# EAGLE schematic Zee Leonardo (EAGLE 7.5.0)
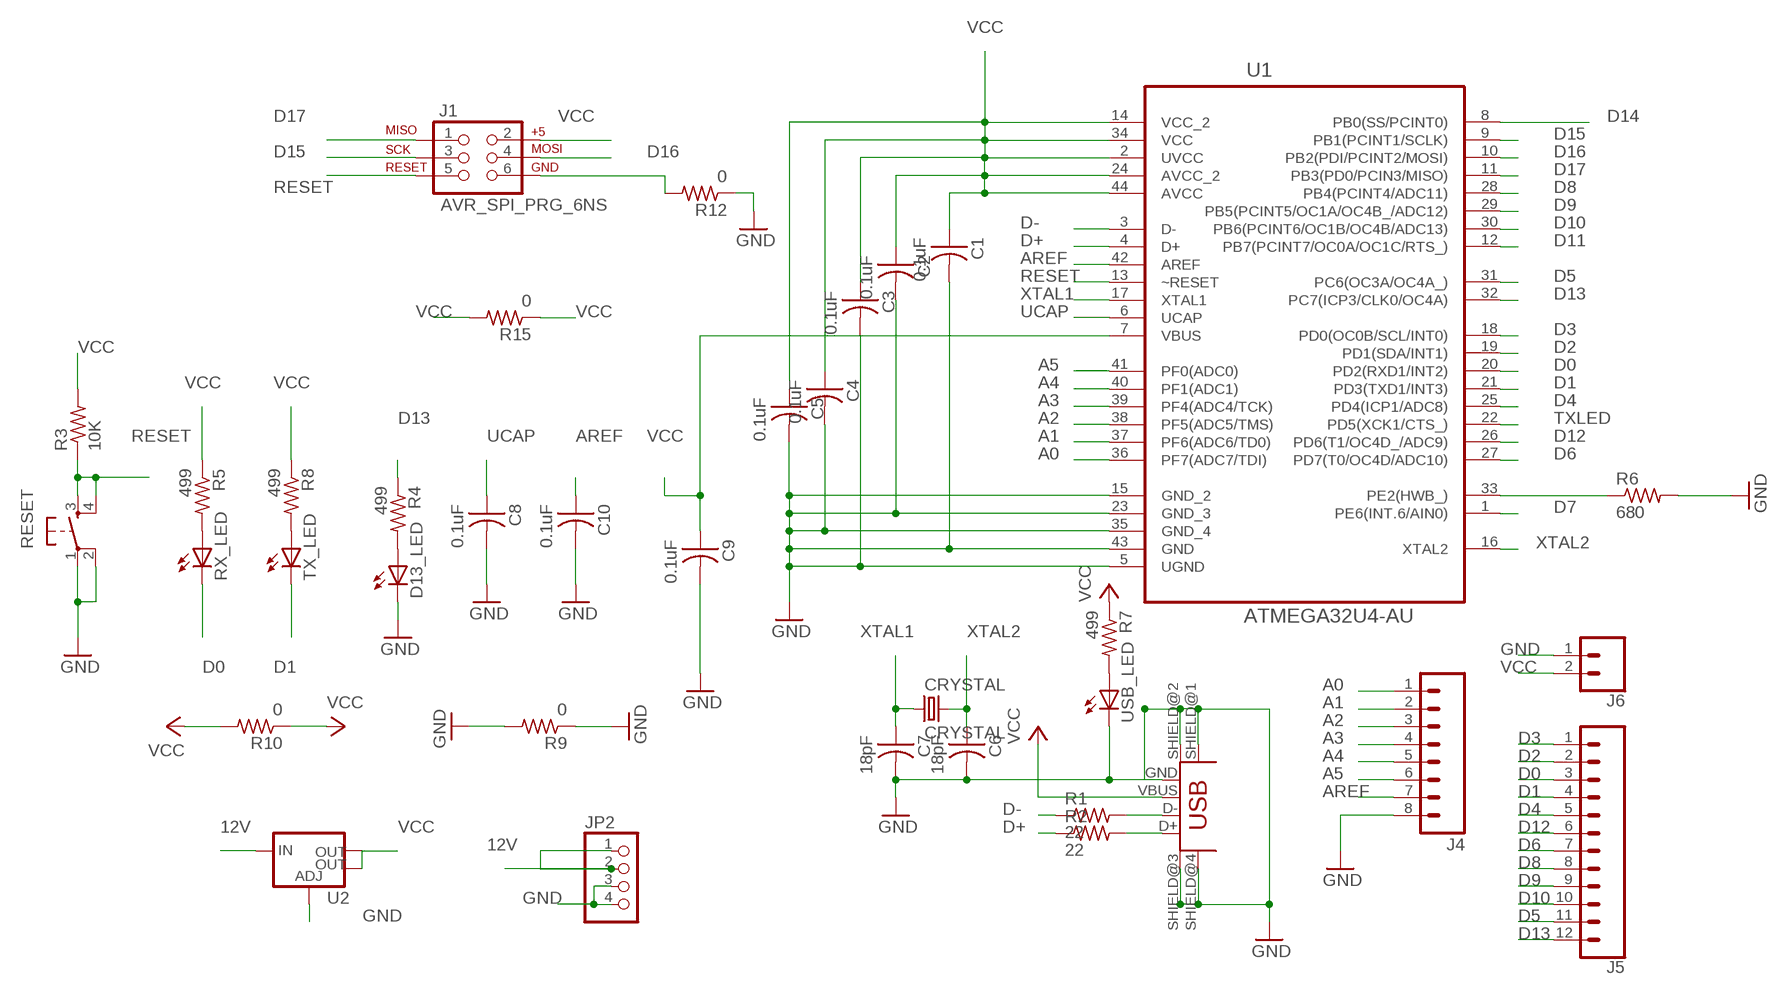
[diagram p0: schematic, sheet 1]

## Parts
C1  0.1uF  CAP-US1206FAB  [C1206FAB]
C2  0.1uF  CAP-US1206FAB  [C1206FAB]
C3  0.1uF  CAP-US1206FAB  [C1206FAB]
C4  0.1uF  CAP-US1206FAB  [C1206FAB]
C5  0.1uF  CAP-US1206FAB  [C1206FAB]
C6  18pF  CAP-US1206FAB  [C1206FAB]
C7  18pF  CAP-US1206FAB  [C1206FAB]
C8  0.1uF  CAP-US1206FAB  [C1206FAB]
C9  0.1uF  CAP-US1206FAB  [C1206FAB]
C10  0.1uF  CAP-US1206FAB  [C1206FAB]
CRYSTAL  CRYSTAL  [2-SMD-5X3MM]
D13_LED  LED1206  [1206]
J1  AVR_SPI_PRG_6NS  [2X3-NS]
J4  M08NO_SILK  [1X08_PIN1_NO_SILK]
J5  CONN_12NO_SILK  [1X12_NO_SILK]
J6  CONN_021X02_NO_SILK  [1X02_NO_SILK]
JP2  PINHD-1X4  [1X04]
R1  22  RES-US1206FAB  [R1206FAB]
R2  22  RES-US1206FAB  [R1206FAB]
R3  10K  RES-US1206FAB  [R1206FAB]
R4  499  RESISTOR1206  [1206]
R5  499  RESISTOR1206  [1206]
R6  680  RES-US1206FAB  [R1206FAB]
R7  499  RESISTOR1206  [1206]
R8  499  RESISTOR1206  [1206]
R9  0  RES-US1206FAB  [R1206FAB]
R10  0  RES-US1206FAB  [R1206FAB]
R12  0  RES-US1206FAB  [R1206FAB]
R15  0  RES-US1206FAB  [R1206FAB]
RESET  6MM_SWITCH6MM_SWITCH  [6MM_SWITCH]
RX_LED  LED1206  [1206]
TX_LED  LED1206  [1206]
U1  ATMEGA32U4-AU  [QFP80P1200X1200X120-44N]
U2  V_REG_LM1117SOT223  [SOT223]
USB_LED  LED1206  [1206]
USB_UPLOAD  USB_MINIB  [USB_MINIB]

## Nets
12V: JP2.1 JP2.2 U2.3(IN)
A0: J4.1 U1.36(PF7(ADC7/TDI))
A1: J4.2 U1.37(PF6(ADC6/TD0))
A2: J4.3 U1.38(PF5(ADC5/TMS))
A3: J4.4 U1.39(PF4(ADC4/TCK))
A4: J4.5 U1.40(PF1(ADC1))
A5: J4.6 U1.41(PF0(ADC0))
AREF: C10.1 J4.7 U1.42(AREF)
D0: J5.3 RX_LED.2(C) U1.20(PD2(RXD1/INT2))
D1: J5.4 TX_LED.2(C) U1.21(PD3(TXD1/INT3))
D2: J5.2 U1.19(PD1(SDA/INT1))
D3: J5.1 U1.18(PD0(OC0B/SCL/INT0))
D4: J5.5 U1.25(PD4(ICP1/ADC8))
D5: J5.11 U1.31(PC6(OC3A/OC4A_))
D6: J5.7 U1.27(PD7(T0/OC4D/ADC10))
D7: U1.1(PE6(INT.6/AIN0))
D8: J5.8 U1.28(PB4(PCINT4/ADC11))
D9: J5.9 U1.29(PB5(PCINT5/OC1A/OC4B_/ADC12))
D10: J5.10 U1.30(PB6(PCINT6/OC1B/OC4B/ADC13))
D11: U1.12(PB7(PCINT7/OC0A/OC1C/RTS_))
D12: J5.6 U1.26(PD6(T1/OC4D_/ADC9))
D13: J5.12 R4.1 U1.32(PC7(ICP3/CLK0/OC4A))
D14: U1.8(PB0(SS/PCINT0))
D15: J1.3 U1.9(PB1(PCINT1/SCLK))
D16: J1.4 U1.10(PB2(PDI/PCINT2/MOSI))
D17: J1.1 U1.11(PB3(PD0/PCIN3/MISO))
D+: R2.1 U1.4(D+)
D-: R1.1 U1.3(D-)
GND: C1.2 C2.2 C3.2 C4.2 C5.2 C6.2 C7.2 C8.2 C9.2 C10.2 D13_LED.2(C) J4.8 J6.1 JP2.3 JP2.4 R6.2 R9.1 R9.2 R12.1 RESET.1(P) RESET.2(P1) U1.5(UGND) U1.15(GND_2) U1.23(GND_3) U1.35(GND_4) U1.43(GND) U2.1(ADJ) USB_LED.2(C) USB_UPLOAD.GND USB_UPLOAD.SHIELD@1(SHIELD) USB_UPLOAD.SHIELD@2(SHIELD1) USB_UPLOAD.SHIELD@3(SHIELD2) USB_UPLOAD.SHIELD@4(SHIELD3)
N$1: R1.2 USB_UPLOAD.D-
N$2: R2.2 USB_UPLOAD.D+
N$3: D13_LED.1(A) R4.2
N$4: R5.2 RX_LED.1(A)
N$5: R7.2 USB_LED.1(A)
N$6: R8.2 TX_LED.1(A)
N$13: J1.6 R12.2
N$35: R6.1 U1.33(PE2(HWB_))
RESET: J1.5 R3.1 RESET.3(S) RESET.4(S1) U1.13(~RESET)
TXLED: U1.22(PD5(XCK1/CTS_))
UCAP: C8.1 U1.6(UCAP)
VCC: C1.1 C2.1 C3.1 C4.1 C5.1 C9.1 J1.2 J6.2 R3.2 R5.1 R7.1 R8.1 R10.1 R10.2 R15.1 R15.2 U1.2(UVCC) U1.7(VBUS) U1.14(VCC_2) U1.24(AVCC_2) U1.34(VCC) U1.44(AVCC) U2.2(OUT) U2.4(OUT) USB_UPLOAD.VBUS
XTAL1: C7.1 CRYSTAL.P$1 U1.17(XTAL1)
XTAL2: C6.1 CRYSTAL.P$2 U1.16(XTAL2)

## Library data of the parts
C1-C10 = fab:CAP-US
CRYSTAL = fab:CRYSTAL
D13_LED RX_LED TX_LED USB_LED = ng:LED
J1 = SparkFun-ConnectorsModified:AVR_SPI_PRG_6: AVR ISP 6 Pin This is the reduced ISP connector for AVR programming. Common on Arduino. This footprint will take up less PCB space and can be used with a 10-pin to 6-pin adapter such as SKU: BOB-08508 **Special note about "TEST_POINT" package. The stop mask is on the top side, so if you want your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
J4 = SparkFun-ConnectorsModified:M08: Header 8 Standard 8-pin 0.1" header. Use with straight break away headers (SKU : PRT-00116), right angle break away headers (PRT-00553), swiss pins (PRT-00743), machine pins (PRT-00117), and female headers (PRT-00115).
J5 = SparkFun-Connectors:CONN_12: Multi connection point. Often used as Generic Header-pin footprint for 0.1 inch spaced/style header connections On any of the 0.1 inch spaced packages, you can populate with these: Break Away Headers - Straight (PRT-00116) Break Away Male Headers - Right Angle (PRT-00553) Female Headers (PRT-00115)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
J6 = SparkFun-Connectors:CONN_02: Multi connection point. Often used as Generic Header-pin footprint for 0.1 inch spaced/style header connections
JP2 = pinhead:PINHD-1X4: PIN HEADER
R1-R3 R6 R9 R10 R12 R15 = fab:RES-US: Resistor (US Symbol)
R4 R5 R7 R8 = ng:RESISTOR
RESET = fab:6MM_SWITCH: OMRON SWITCH
U1 = Atmel_By_element14_Batch_1:ATMEGA32U4-AU: 8-bit Microcontroller with ISP Flash and USB Controller; MPN: ATMEGA32U4-AU; OC_FARNELL: 1748525; OC_NEWARK: 26R5633; PACKAGE: TQFP-44; SUPPLIER: Atmel
U2 = fab:V_REG_LM1117: Voltage Regulator LM1117 Standard adjustable voltage regulator but in SMD form. Spark Fun Electronics SKU : COM-00595; PROD_ID: VREG-08170
USB_UPLOAD = fab:USB_MINIB

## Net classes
0 default: width 0.305 mm, drill 0.305 mm, clearance 0.305 mm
